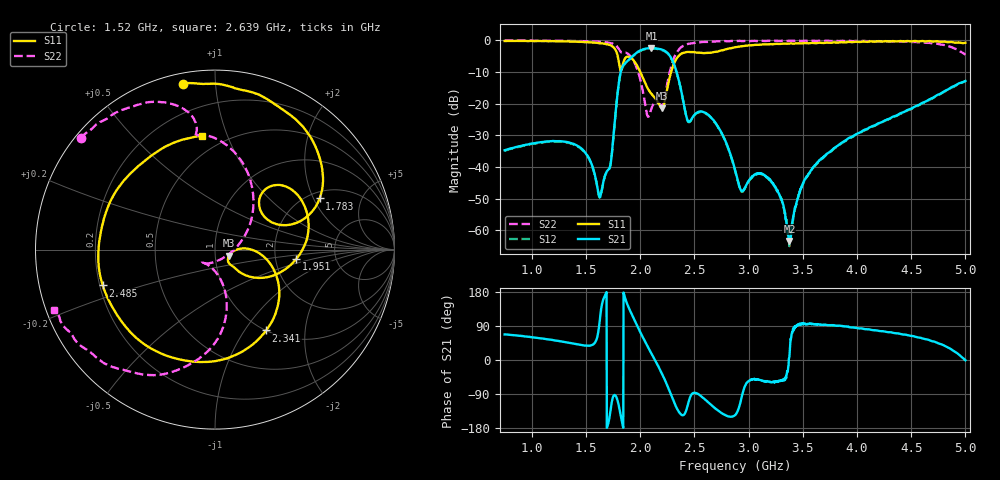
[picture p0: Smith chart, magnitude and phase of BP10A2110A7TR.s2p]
!Agilent Technologies,E8358A,US41080443,A.07.50.56
!Agilent E8358A: A.07.50.56
!Date: Friday, August 07, 2015 14:22:22
!Correction: S11(Full 2 Port(1,2))
!S21(Full 2 Port(1,2))
!S12(Full 2 Port(1,2))
!S22(Full 2 Port(1,2))
!S2P File: Measurements: S11, S21, S12, S22:
# Hz S  dB  R 50
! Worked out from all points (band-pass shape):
!   1601 points, 750 MHz to 5 GHz, reference 50 ohm
!   highest |S21| = -2.41 dB at 2.105 GHz (marker M1); lowest = -63.4 dB at 3.377 GHz (marker M2)
!   |S21| within 3 dB of the highest: 1.916 GHz to 2.284 GHz (367.9 MHz wide, 17.5 % of centre)
!   lowest |S11| = -21.4 dB at 2.203 GHz (marker M3), VSWR 1.19, Z = 58.3 - j4.01 ohm
!   |S11| at or under -10 dB: 2.002 GHz to 2.285 GHz (283.6 MHz wide, 13.2 % of centre)
!   |S22| runs from -24.1 to 0.0 dB; largest |S21 - S12| = 0.012
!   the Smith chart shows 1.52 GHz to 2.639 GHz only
!   S11 on the Smith chart (normalised r, x): 1.52 GHz: 0.05, +0.82; 1.783 GHz: 2.27, +2.24; 1.951 GHz: 2.63, -0.34; 2.341 GHz: 1.00, -1.26; 2.485 GHz: 0.21, -0.15; 2.639 GHz: 0.38, +0.82
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7.5e8  -0.16 151.9  -34.72 67.5  -34.85 67.6  -0.01 166.4
1.459219e9  -0.41 108.7  -34.15 39.3  -34.29 39.4  -0.18 144.0
1.520312e9  -0.53 100.9  -36.74 37.7  -36.88 38.1  -0.27 140.2
1.637188e9  -0.90 80.0  -48.83 127.2  -48.90 128.2  -0.47 129.9
1.7275e9  -1.52 53.7  -39.04 -131.7  -39.16 -131.5  -0.81 117.0
1.783281e9  -3.75 26.0  -19.46 -99.6  -19.62 -99.3  -1.77 103.6
1.857656e9  -5.85 44.9  -7.30 167.1  -7.44 167.3  -3.82 97.9
1.950625e9  -6.81 -6.4  -4.34 103.7  -4.46 103.7  -7.17 63.5
2.104688e9  -16.89 -42.9  -2.41 16.8  -2.54 16.9  -21.47 -114.7
2.168438e9  -19.81 -43.1  -2.60 -17.0  -2.72 -17.0  -19.79 -135.2
2.202969e9  -21.42 -23.7  -2.90 -36.9  -3.03 -36.8  -20.46 -112.6
2.341094e9  -5.46 -57.7  -10.55 -128.9  -10.69 -128.7  -3.61 -102.9
2.484531e9  -3.65 -162.3  -24.26 -87.9  -24.42 -87.8  -0.85 -142.0
2.638594e9  -3.91 96.6  -23.82 -114.3  -23.89 -114.2  -0.35 -159.4
2.760781e9  -3.07 26.4  -29.90 -141.9  -29.99 -141.3  -0.26 -167.4
2.875e9  -2.14 -22.6  -40.84 -145.7  -41.01 -145.7  -0.22 -173.5
3.204375e9  -1.17 -101.5  -44.28 -58.1  -44.41 -58.4  -0.11 174.5
3.377031e9  -0.94 -122.5  -63.38 9.9  -65.04 10.7  -0.07 169.8
3.584219e9  -0.77 -139.4  -40.77 95.5  -40.79 95.5  -0.07 163.5
4.293438e9  -0.33 -164.0  -24.79 73.3  -24.94 73.4  -0.31 137.2
4.800781e9  -0.33 180.0  -16.13 38.6  -16.26 38.5  -1.40 91.8
5e9  -0.74 172.1  -12.81 -0.7  -12.96 -1.1  -4.48 18.6
